|//////////////////////////////////////////////////////////////////////////////
|//////////////////////////////////////////////////////////////////////////////
|   @@@@@@@   @@@@@@@   @@@@@@@   @@@@@@@   @@@@@@@   @@@@@@   @@
|   @@@@@@@@@   @@@@@@@@@   @@@@@@@@@   @@@@@@@@@   @@@@@@@@@ @@@@@@@@  @
|   @@@   @@@ @@@   @@@ @@@   @@@   @@@ @@@   @@@@   @@@  @
|   @@   @@ @@   @@ @@@@@@@@@@@ @@@@@@@@@@@ @@   @@   @@ @@
|   @@@   @@@ @@   @@   @@@ @@@   @@   @@   @@ @@
|   @@@@@@@@@  @@   @@  @@@@@@@@@   @@@@@@@@@  @@   @@   @@ @@
|   @@@@@@@   @@   @@   @@@@@@@   @@@@@@@   @@   @@   @@ @@
|   IBIS Model of MC74VHC1G50
|   Single Non-Inverting Buffer
|   Package Type: SC-74A, CASE 318BQ (DBV)
|   SC-88A/SC-70-5, CASE 419A-02 (DF)
|   SOT-953, CASE 527AE (P5)
|   SOT-553 (XV5), CASE 463B-01
|   UDFN6, CASE 517AQ (1.45 x 1.00 mm)
|   UDFN6, CASE 517BX (1.00 x 1.00 mm)
|   The model is covering the following Vccs:
|   2.0V, 2.5V, 3.3V, 5.0V
|//////////////////////////////////////////////////////////////////////////////
|//////////////////////////////////////////////////////////////////////////////
[IBIS Ver]   3.2
|   7.2 compatible
|//////////////////////////////////////////////////////////////////////////////
[Comment Char] |_char
|//////////////////////////////////////////////////////////////////////////////
[File Name]   74vhc1g50_va_r0.ibs
|//////////////////////////////////////////////////////////////////////////////
[File Rev]   0.0
|   0.0 - February 06, 2025 - File created
|//////////////////////////////////////////////////////////////////////////////
[Date]   Feb 06, 2025
|//////////////////////////////////////////////////////////////////////////////
[Source]   From lab measurements and simulations at onsemi
|//////////////////////////////////////////////////////////////////////////////
[Notes]
   - The currents greater than +/- 100 mA are extrapolated
|//////////////////////////////////////////////////////////////////////////////
[Disclaimer]
   - onsemi Corporation hereby grants
   the user of this IBIS model a license to use this model
   under the following terms. This license is nonexclusive
   and nontransferable. Before using this IBIS model.
   After reading the terms and conditions of this license,
   the user either must accept these terms,
   or the IBIS model should be returned to onsemi within 30 days.
   - The user is hereby granted a license to use the IBIS model.
   This shall not be construed as a right to sell,
   or otherwise profit either by leasing or renting this software.
   - The user may modify the IBIS model to suit his specific
   applications but rights to derivative works and such
   modifications shall belong to onsemi.
   - This IBIS model is provided on an "as is" basis.
   onsemi makes absolutely no warranty with respect
   to the information contained herein.
   By use of this IBIS model, the user assumes full risk as to the
   quality and suitablility of the model to his particular use,
   and by using this model assumes the entire risk.
   Under all circumstances the user shall not hold
   onsemi liable in any way for the results obtained.
   onsemi reserves the right to make to improve
   the model for reliability, function, or design.
   onsemi does not convey any license under patent
   rights or any other intellectual property rights,
   including those of third parties.
   - onsemi is not obligated to provide maintenance
   or support for the licensed IBIS model.
   - Cont onsemi at ATTN:LOGIC APPLICATIONS/IBIS MODEL.
   5701 N Pima Rd, Scottsdale, AZ 85250
|//////////////////////////////////////////////////////////////////////////////
[Copyright]   (c) 2025 onsemi Corp.
|//////////////////////////////////////////////////////////////////////////////
|//////////////////////////////////////////////////////////////////////////////
[Component]   MC74VHC1G50DBVT1G
|//////////////////////////////////////////////////////////////////////////////
[Manufacturer]  onsemi
|   Data Sheet:   MC74VHC1G50/D , Rev. 20,  Apr, 2023
|//////////////////////////////////////////////////////////////////////////////
[Package]
|   SC-74A
| DBV SUFFIX
| CASE 318BQ
| variable   typ   min   max
R_pkg   0.0710   0.0522   0.0935
L_pkg   1.2331nH   1.0634nH   1.4484nH
C_pkg   0.1280pF   0.1167pF   0.1367pF
|//////////////////////////////////////////////////////////////////////////////
[Pin]   signal_name   model_name   R_pin   L_pin   C_pin
1   NC   NC   0.0522   1.0634nH   0.1235pF
2   A   In   0.0588   1.1995nH   0.1367pF
3   GND   GND   0.0828   1.3327nH   0.1351pF
4   Y   Out   0.0935   1.4484nH   0.1279pF
5   VCC   POWER   0.0679   1.1215nH   0.1167pF
|//////////////////////////////////////////////////////////////////////////////
|//////////////////////////////////////////////////////////////////////////////
[Component]   MC74VHC1G50DFT1G
|//////////////////////////////////////////////////////////////////////////////
[Manufacturer]  onsemi
|   Data Sheet:   MC74VHC1G50/D , Rev. 20,  Apr, 2023
|//////////////////////////////////////////////////////////////////////////////
[Package]
| SC-88A / SC-70-5
|   DF SUFFIX
|   CASE 419A-02
| variable   typ   min   max
R_pkg   0.0201   0.0170   0.0250
L_pkg   0.9982nH   0.8810nH   1.0690nH
C_pkg   0.1466pF   0.1187pF   0.2051pF
|//////////////////////////////////////////////////////////////////////////////
[Pin]   signal_name   model_name   R_pin   L_pin   C_pin
1   NC   NC   0.0191   1.0690nH   0.1625pF
2   A   In   0.0187   0.8810nH   0.1217pF
3   GND   GND   0.0170   1.0315nH   0.2051pF
4   Y   Out   0.0207   0.9600nH   0.1249pF
5   VCC   POWER   0.0250   1.0497nH   0.1187pF
|//////////////////////////////////////////////////////////////////////////////
|//////////////////////////////////////////////////////////////////////////////
[Component]   MC74VHC1G50DFT2G
|//////////////////////////////////////////////////////////////////////////////
[Manufacturer]  onsemi
|   Data Sheet:   MC74VHC1G50/D , Rev. 20,  Apr, 2023
|//////////////////////////////////////////////////////////////////////////////
[Package]
R_pkg   0.0201   0.0170   0.0250
L_pkg   0.9982nH   0.8810nH   1.0690nH
C_pkg   0.1466pF   0.1187pF   0.2051pF
|//////////////////////////////////////////////////////////////////////////////
[Pin]   signal_name   model_name   R_pin   L_pin   C_pin
1   NC   NC   0.0191   1.0690nH   0.1625pF
2   A   In   0.0187   0.8810nH   0.1217pF
3   GND   GND   0.0170   1.0315nH   0.2051pF
4   Y   Out   0.0207   0.9600nH   0.1249pF
5   VCC   POWER   0.0250   1.0497nH   0.1187pF
|//////////////////////////////////////////////////////////////////////////////
|//////////////////////////////////////////////////////////////////////////////
[Component]   MC74VHC1G50DFT2G-Q
|//////////////////////////////////////////////////////////////////////////////
[Manufacturer]  onsemi
|   Data Sheet:   MC74VHC1G50/D , Rev. 20,  Apr, 2023
|//////////////////////////////////////////////////////////////////////////////
[Package]
R_pkg   0.0201   0.0170   0.0250
L_pkg   0.9982nH   0.8810nH   1.0690nH
C_pkg   0.1466pF   0.1187pF   0.2051pF
|//////////////////////////////////////////////////////////////////////////////
[Pin]   signal_name   model_name   R_pin   L_pin   C_pin
1   NC   NC   0.0191   1.0690nH   0.1625pF
2   A   In   0.0187   0.8810nH   0.1217pF
3   GND   GND   0.0170   1.0315nH   0.2051pF
4   Y   Out   0.0207   0.9600nH   0.1249pF
5   VCC   POWER   0.0250   1.0497nH   0.1187pF
|//////////////////////////////////////////////////////////////////////////////
|//////////////////////////////////////////////////////////////////////////////
[Component]   MC74VHC1G50P5T5G
|//////////////////////////////////////////////////////////////////////////////
[Manufacturer]  onsemi
|   Data Sheet:   MC74VHC1G50/D , Rev. 20,  Apr, 2023
|//////////////////////////////////////////////////////////////////////////////
[Package]
|  SOT-953
| P5  SUFFIX
| CASE 527AE
| variable   typ   min   max
R_pkg   0.0786   0.0731   0.0817
L_pkg   1.1377nH   1.0330nH   1.1757nH
C_pkg   0.0487pF   0.0295pF   0.0642pF
|//////////////////////////////////////////////////////////////////////////////
[Pin]   signal_name   model_name   R_pin   L_pin   C_pin
1   A   In   0.0817   1.1757nH   0.0433pF
2   GND   GND   0.0731   1.0330nH   0.0295pF
3   NC   NC   0.0805   1.1531nH   0.0500pF
4   Y   Out   0.0789   1.1637nH   0.0642pF
5   VCC   POWER   0.0787   1.1630nH   0.0567pF
|//////////////////////////////////////////////////////////////////////////////
|//////////////////////////////////////////////////////////////////////////////
[Component]   MC74VHC1G50MU1TCG
|//////////////////////////////////////////////////////////////////////////////
[Manufacturer]  onsemi
|   Data Sheet:   MC74VHC1G50/D , Rev. 20,  Apr, 2023
|//////////////////////////////////////////////////////////////////////////////
[Package]
|   UDFN-6
| 1.45 x 1.0
| CASE 517AQ
| variable   typ   min   max
R_pkg   0.0499   0.0010   0.0568
L_pkg   0.4063nH   0.0145nH   0.4786nH
C_pkg   0.1074pF   0.0765pF   0.1119pF
|//////////////////////////////////////////////////////////////////////////////
[Pin]   signal_name   model_name   R_pin   L_pin   C_pin
1   NC   NC   0.0568   0.4786nH   0.1119pF
2   A   In   0.0469   0.3812nH   0.1077pF
3   GND   GND   0.0541   0.4521nH   0.1099pF
4   Y   Out   0.0513   0.4206nH   0.1072pF
5   NC   NC   0.0010   0.0145nH   0.0765pF
6   VCC   POWER   0.0484   0.3921nH   0.1051pF
|//////////////////////////////////////////////////////////////////////////////
|//////////////////////////////////////////////////////////////////////////////
[Component]   MC74VHC1G50MU3TCG
|//////////////////////////////////////////////////////////////////////////////
[Manufacturer]  onsemi
|   Data Sheet:   MC74VHC1G50/D , Rev. 20,  Apr, 2023
|//////////////////////////////////////////////////////////////////////////////
[Package]
|  UDFN-6
| 1.0 x 1.0
| CASE 517BX
| variable   typ   min   max
R_pkg   0.0419   0.0344   0.0490
L_pkg   0.4237nH   0.3470nH   0.5107nH
C_pkg   0.1104pF   0.1061pF   0.1153pF
|//////////////////////////////////////////////////////////////////////////////
[Pin]   signal_name   model_name   R_pin   L_pin   C_pin
1   NC   NC   0.0421   0.4133nH   0.1099pF
2   A   In   0.0344   0.3470nH   0.1061pF
3   GND   GND   0.0443   0.4580nH   0.1121pF
4   Y   Out   0.0490   0.5107nH   0.1153pF
5   NC   NC   0.0004   0.0379nH   0.0765pF
6   VCC   POWER   0.0438   0.4489nH   0.1118pF
|//////////////////////////////////////////////////////////////////////////////
|//////////////////////////////////////////////////////////////////////////////
[Component]   MC74VHC1G50XV5T2G
|//////////////////////////////////////////////////////////////////////////////
[Manufacturer]  onsemi
|   Data Sheet:   MC74VHC1G50/D , Rev. 20,  Apr, 2023
|//////////////////////////////////////////////////////////////////////////////
[Package]
|  SOT-553
| XV5 SUFFIX
| CASE 463B-01
| variable   typ   min   max
R_pkg   0.0321   0.0287   0.0357
L_pkg   0.9169nH   0.7230nH   1.1357nH
C_pkg   0.2220pF   0.1035pF   0.3741pF
|//////////////////////////////////////////////////////////////////////////////
[Pin]   signal_name   model_name   R_pin   L_pin   C_pin
1   NC   NC   0.0341   0.7230nH   0.1035pF
2   A   In   0.0287   0.8933nH   0.2377pF
3   GND   GND   0.0290   1.0725nH   0.3741pF
4   Y   Out   0.0357   0.7602nH   0.1139pF
5   VCC   POWER   0.0330   1.1357nH   0.2807pF
|//////////////////////////////////////////////////////////////////////////////
|//////////////////////////////////////////////////////////////////////////////
[Model Selector]   In
In_20   Vcc = 2.00
In_25   Vcc = 2.50
In_33   Vcc = 3.30
In_50   Vcc = 5.00
|//////////////////////////////////////////////////////////////////////////////
[Model Selector]   Out
Out_20   Vcc = 2.00
Out_25   Vcc = 2.50
Out_33   Vcc = 3.30
Out_50   Vcc = 5.00
| Models and submodels in the file (8): In_20 (Input), Out_20 (Output), In_25 (Input), Out_25 (Output), In_33 (Input), Out_33 (Output), In_50 (Input), Out_50 (Output)
